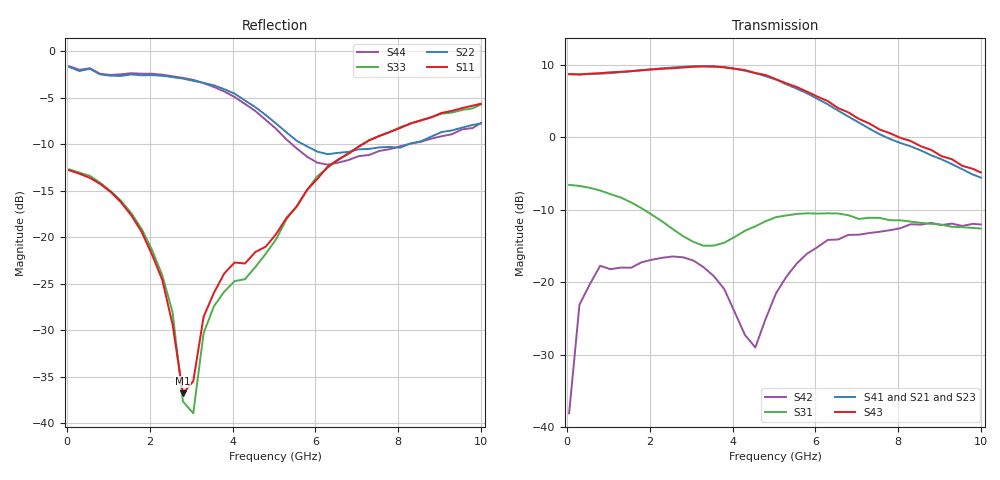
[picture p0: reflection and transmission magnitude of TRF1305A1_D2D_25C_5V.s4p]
! Created Tue Jun 24 22:54:00 2025
# hz S ma R 50
! 4 Port Network Data from SP1.SP block
! PORT[1] = INP
! PORT[2] = OUTM
! PORT[3] = INM
! PORT[4] = OUTP
! freq  magS11  angS11  magS12  angS12  magS13  angS13  magS14  angS14
!  magS21  angS21  magS22  angS22  magS23  angS23  magS24  angS24
!  magS31  angS31  magS32  angS32  magS33  angS33  magS34  angS34
!  magS41  angS41  magS42  angS42  magS43  angS43  magS44  angS44
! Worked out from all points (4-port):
!   41 points, 50 MHz to 10 GHz, reference 50 ohm
!   strongest paths, dB at 50 MHz, 2.55 GHz, 5.05 GHz, 7.55 GHz, 10 GHz:
!     S43: 8.7, 9.5, 8.0, 1.1, -4.9
!     S41: 8.7, 9.6, 8.0, 0.4, -5.6
!     S21: 8.8, 9.4, 7.8, 0.6, -5.1
!     S23: 8.9, 9.4, 7.6, 0.6, -5.0
!     S31: -6.6, -12.7, -11.0, -11.1, -12.6
!     S42: -38.1, -16.5, -21.5, -13.0, -12.0
!   lowest |S11| = -36.8 dB at 2.8 GHz (marker M1), VSWR 1.03, Z = 48.7 - j0.486 ohm
!   |S11| at or under -10 dB: start of sweep to 7.144 GHz
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5e7  0.2292 -1.6  0.002442 -6.9  0.476 -2.0  0.002153 49.5
     2.761 178.0  0.8245 178.5  2.771 -2.0  0.01138 120.6
     0.4693 -2.4  0.001007 143.6  0.2319 -2.5  0.001131 94.8
     2.724 -2.1  0.01242 131.9  2.732 177.7  0.8316 178.8
1.8e9  0.1071 -73.0  0.03318 6.6  0.3278 -77.3  0.02287 -2.2
       2.887 105.3  0.743 140.2  2.884 -73.3  0.132 13.4
       0.324 -77.3  0.02427 -6.1  0.1111 -71.6  0.03221 14.2
       2.909 -71.5  0.1371 11.9  2.902 106.9  0.7578 143.8
2.8e9  0.01448 -159.8  0.04282 -17.9  0.2081 -136.3  0.02613 -42.5
       2.984 60.1  0.7127 115.9  2.998 -119.4  0.143 -12.8
       0.208 -137.6  0.02798 -47.4  0.01308 -137.6  0.04309 -16.0
       3.067 -116.8  0.1485 -17.3  3.033 61.3  0.7194 120.8
4.05e9  0.07311 59.7  0.05209 -50.0  0.2054 121.8  0.02435 -89.7
        2.895 -2.3  0.5915 85.4  2.888 178.6  0.05245 -68.0
        0.205 119.1  0.02522 -92.9  0.05803 62.6  0.05344 -51.2
        2.978 179.3  0.06218 -85.4  2.979 -0.7  0.5675 89.8
5.3e9  0.1269 58.3  0.05498 -88.6  0.2908 56.6  0.01589 -121.4
       2.286 -67.3  0.3669 65.9  2.257 112.7  0.1012 85.3
       0.2888 53.0  0.01496 -128.2  0.1247 64.9  0.057 -88.4
       2.322 114.5  0.109 96.5  2.36 -65.0  0.3359 73.9
6.8e9  0.2809 34.5  0.0497 -132.2  0.2988 13.1  0.0112 -134.8
       1.374 -131.4  0.2876 78.1  1.394 48.2  0.2005 41.9
       0.2898 12.0  0.0116 -135.0  0.2841 36.8  0.05181 -125.7
       1.39 47.6  0.2121 44.2  1.486 -129.5  0.2601 89.1
1e10  0.5224 -36.0  0.03832 158.8  0.2379 -29.0  0.005441 159.4
      0.5557 125.5  0.4086 68.6  0.5619 -61.6  0.2475 -7.5
      0.2346 -26.9  0.01146 165.2  0.5172 -33.6  0.03887 165.2
      0.5269 -59.1  0.2501 -5.2  0.5715 126.0  0.4115 73.3
